FUNCTION_BLOCK "Bool1"
VERSION : 0.1
   VAR_INPUT
      in1 : Bool;
      in2 : Bool;
      in3 : Bool;
   END_VAR

   VAR_OUTPUT
      out1 : Bool;
   END_VAR


BEGIN
NETWORK
TITLE =
      SET;
      A #in1;
      O(;
      A #in2;
      AN #in3;
      );
      = #out1;

END_FUNCTION_BLOCK

